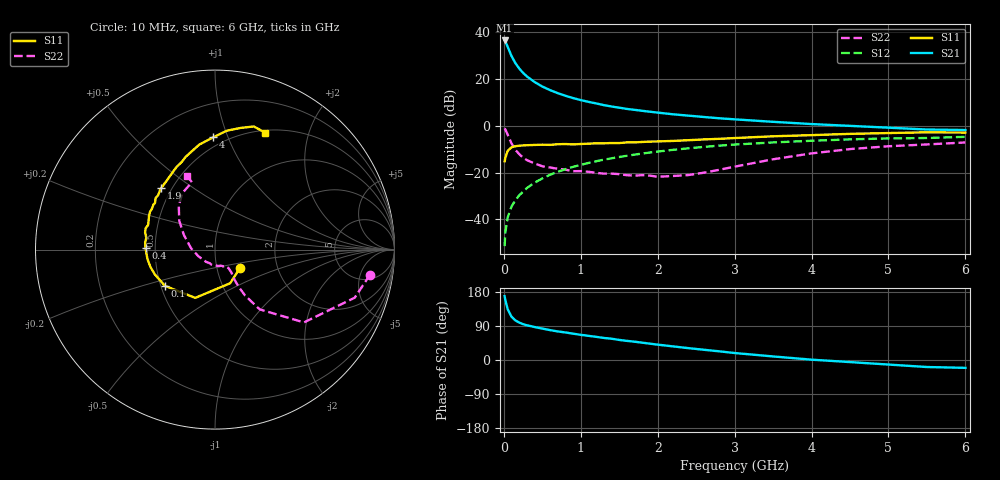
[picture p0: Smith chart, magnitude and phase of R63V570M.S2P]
! SIEMENS Small Signal Semiconductors
! BFR193
! Si NPN RF Bipolar Junction Transistor in SOT23
! VCE = 3.5 V  IC = 70 mA
! Common Emitter S-Parameters:  May  1996
# GHz  S  MA  R  50
!  f  S11  S21  S12  S22
! GHz  MAG  ANG  MAG  ANG  MAG  ANG  MAG  ANG
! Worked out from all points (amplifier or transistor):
!   36 points, 10 MHz to 6 GHz, reference 50 ohm
!   highest |S21| = 36.3 dB at 10 MHz (marker M1)
!   |S21| within 3 dB of that: start of sweep to 53.69 MHz
!   unconditionally stable (mu >= 1): 314.8 MHz to 1.871 GHz
!   at 250 MHz: K = 0.99, MSG = 25.3 dB, |S12| = -28.2 dB
!   at 1.4 GHz: K = 1.02, MAG = 10.1 dB, |S12| = -13.9 dB
!   at 6 GHz: K = 0.96, MSG = 1.4 dB, |S12| = -4.8 dB
!   S11 on the Smith chart (normalised r, x): 10 MHz: 1.29, -0.28; 100 MHz: 0.53, -0.24; 400 MHz: 0.44, +0.01; 1.9 GHz: 0.44, +0.38; 4 GHz: 0.43, +0.89; 6 GHz: 0.53, +1.38
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0.01  0.1729 -36.9  65.03 168.4  0.0027 80.7  0.8751 -9.2
0.02  0.2055 -65.6  61.77 157.6  0.0054 73.7  0.8232 -19.0
0.05  0.2905 -112.2  47.61 134.0  0.0111 71.6  0.6406 -39.3
0.1  0.3446 -144.1  30.19 114.3  0.0189 70.3  0.4162 -53.2
0.15  0.3628 -157.7  21.4 104.4  0.0256 72.5  0.3048 -56.8
0.2  0.3728 -165.2  16.44 98.8  0.0328 73.6  0.2461 -57.5
0.25  0.3781 -170.6  13.25 94.6  0.039 74.9  0.2077 -57.2
0.3  0.3815 -174.7  11.15 91.6  0.0468 76.0  0.1839 -56.3
0.4  0.3869 178.9  8.462 87.0  0.0609 75.8  0.1557 -54.3
0.5  0.3912 174.2  6.787 82.9  0.0747 75.4  0.1362 -54.0
0.6  0.3882 170.2  5.696 78.9  0.0895 74.5  0.128 -53.8
0.7  0.4004 166.5  4.916 75.4  0.1035 73.6  0.1203 -55.2
0.9  0.3971 159.8  3.857 69.5  0.1321 70.9  0.1067 -58.5
1.1  0.412 153.2  3.199 63.8  0.1599 68.2  0.1039 -64.5
1.5  0.4238 142.0  2.408 53.0  0.2143 62.3  0.0924 -80.3
1.9  0.4554 131.4  1.971 43.1  0.2669 56.2  0.0859 -104.2
2.2  0.4714 124.2  1.739 35.9  0.3042 51.4  0.0844 -126.2
3.5  0.5911 98.6  1.202 9.4  0.4377 30.5  0.1915 154.8
4  0.6259 90.9  1.077 0.9  0.4753 23.4  0.2557 141.2
4.5  0.6659 84.3  0.986 -5.5  0.5083 16.3  0.3156 129.7
5.5  0.7194 72.5  0.824 -18.5  0.5432 2.5  0.3966 108.9
6  0.7088 66.8  0.804 -20.7  0.5763 -1.4  0.4369 110.6
